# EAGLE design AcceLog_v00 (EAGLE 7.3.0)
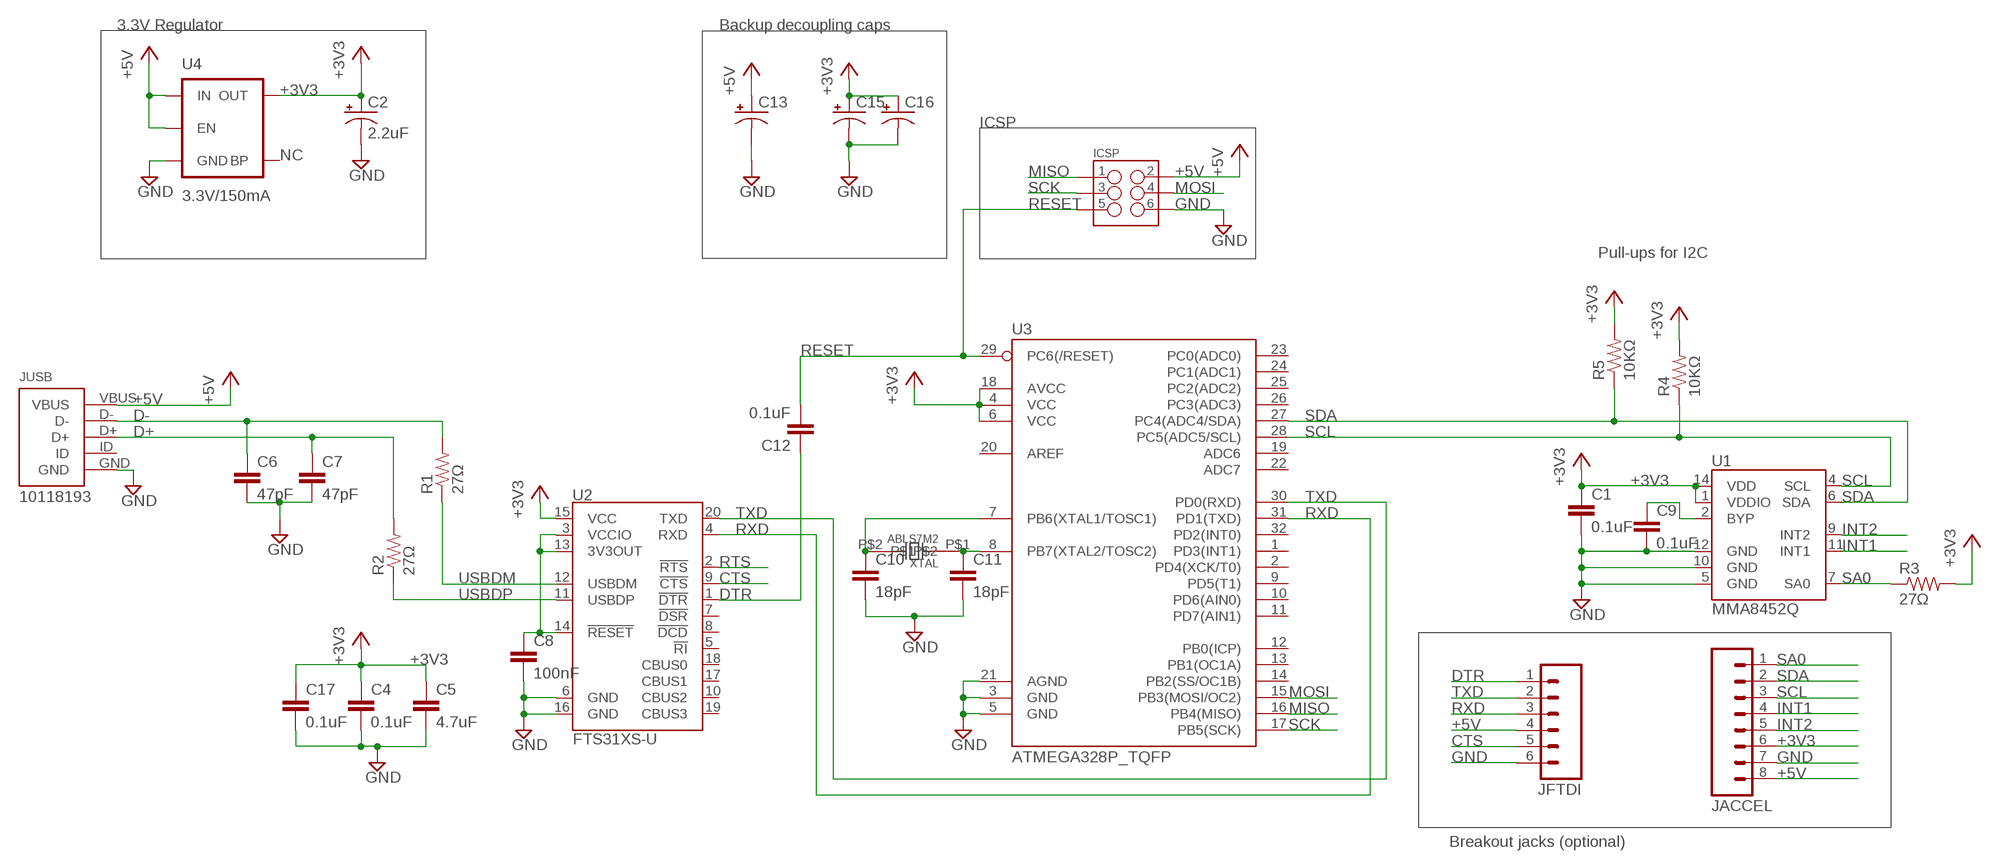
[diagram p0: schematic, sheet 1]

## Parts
C1  0.1uF  CAP0603-CAP  [0603-CAP]
C2  2.2uF  CAP_POL1206  [EIA3216]
C4  0.1uF  CAP0603-CAP  [0603-CAP]
C5  4.7uF  CAP0603-CAP  [0603-CAP]
C6  47pF  CAP0603-CAP  [0603-CAP]
C7  47pF  CAP0603-CAP  [0603-CAP]
C8  100nF  CAP0603-CAP  [0603-CAP]
C9  0.1uF  CAP0603-CAP  [0603-CAP]
C10  18pF  CAP0603-CAP  [0603-CAP]
C11  18pF  CAP0603-CAP  [0603-CAP]
C12  0.1uF  CAP0603-CAP  [0603-CAP]
C13  CPOL-USE2-5  [E2-5]
C15  CPOL-USE2-5  [E2-5]
C16  CPOL-USE2-5  [E2-5]
C17  0.1uF  CAP0603-CAP  [0603-CAP]
ICSP  M03X22X3_SILK_MALE_PTH  [2X3]
JACCEL  M08LOCK  [1X08_LOCK]
JFTDI  M06LOCK  [1X06_LOCK]
JUSB  10118193  [10118193]
R1  27Ω  RESISTOR0603-RES  [0603-RES]
R2  27Ω  RESISTOR0603-RES  [0603-RES]
R3  27Ω  RESISTOR0603-RES  [0603-RES]
R4  10KΩ  RESISTOR0603-RES  [0603-RES]
R5  10KΩ  RESISTOR0603-RES  [0603-RES]
U1  MMA8452Q  [QFN-16_0.5MM]
U2  FTS31XS-U  FT231XS  [SSOP20_L]
U3  ATMEGA328P_TQFP  [TQFP32-08]
U4  3.3V/150mA  V_REG_MIC52053.3V  [SOT23-5]
XTAL  ABLS7M2  [ABLS7M2]

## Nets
+3V3: C1.1 C2.A(+) C4.1 C5.1 C15.+ C16.+ C17.1 JACCEL.6 R3.2 R4.2 R5.2 U1.1(VDDIO) U1.14(VDD) U2.15(VCC) U3.4(VCC) U3.6(VCC) U3.18(AVCC) U4.5(OUT)
+5V: C13.+ ICSP.2 JACCEL.8 JFTDI.4 JUSB.VBUS U4.1(IN) U4.3(EN)
CTS: JFTDI.5 U2.9(!CTS)
D+: C7.1 JUSB.D+ R2.2
D-: C6.1 JUSB.D- R1.2
DTR: C12.1 JFTDI.1 U2.1(!DTR)
FTDI3V3: C8.1 U2.3(VCCIO) U2.13(3V3OUT) U2.14(!RESET)
GND: C1.2 C2.C(-) C4.2 C5.2 C6.2 C7.2 C8.2 C9.2 C10.2 C11.2 C13.- C15.- C16.- C17.2 ICSP.6 JACCEL.7 JFTDI.6 JUSB.GND U1.5(GND) U1.10(GND) U1.12(GND) U2.6(GND) U2.16(GND) U3.3(GND) U3.5(GND) U3.21(AGND) U4.2(GND)
INT1: JACCEL.4 U1.11(INT1)
INT2: JACCEL.5 U1.9(INT2)
MISO: ICSP.1 U3.16(PB4(MISO))
MOSI: ICSP.4 U3.15(PB3(MOSI/OC2))
N$10: C10.1 U3.7(PB6(XTAL1/TOSC1)) XTAL.P$2
N$11: C9.1 U1.2(BYP)
N$12: C11.1 U3.8(PB7(XTAL2/TOSC2)) XTAL.P$1
RESET: C12.2 ICSP.5 U3.29(PC6(/RESET))
RTS: U2.2(!RTS)
RXD: JFTDI.3 U2.4(RXD) U3.31(PD1(TXD))
SA0: JACCEL.1 R3.1 U1.7(SA0)
SCK: ICSP.3 U3.17(PB5(SCK))
SCL: JACCEL.3 R4.1 U1.4(SCL) U3.28(PC5(ADC5/SCL))
SDA: JACCEL.2 R5.1 U1.6(SDA) U3.27(PC4(ADC4/SDA))
TXD: JFTDI.2 U2.20(TXD) U3.30(PD0(RXD))
USBDM: R1.1 U2.12(USBDM)
USBDP: R2.1 U2.11(USBDP)
Unconnected: JUSB.ID U2.5(!RI) U2.7(!DSR) U2.8(!DCD) U2.10(CBUS2) U2.17(CBUS1) U2.18(CBUS0) U2.19(CBUS3) U3.1(PD3(INT1)) U3.2(PD4(XCK/T0)) U3.9(PD5(T1)) U3.10(PD6(AIN0)) U3.11(PD7(AIN1)) U3.12(PB0(ICP)) U3.13(PB1(OC1A)) U3.14(PB2(SS/OC1B)) U3.19(ADC6) U3.20(AREF) U3.22(ADC7) U3.23(PC0(ADC0)) U3.24(PC1(ADC1)) U3.25(PC2(ADC2)) U3.26(PC3(ADC3)) U3.32(PD2(INT0)) U4.4(BP)

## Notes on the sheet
- 3.3V Regulator | Backup decoupling caps
- ICSP
- NC
- Pull-ups for I2C
- Breakout jacks (optional)

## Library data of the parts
C1 C4-C12 C17 = SparkFun-Passives:CAP: Capacitor
C2 = SparkFun-Capacitors:CAP_POL: Capacitor Polarized
C13 C15 C16 = rcl:CPOL-US: POLARIZED CAPACITOR, American symbol
ICSP = SparkFun-Connectors:M03X2: 2x3 .1" header. Shrouded, with keying- CONN-10681 SMT- CONN-11415 Pogo pins- HW-11044; PROD_ID: CONN-09701
JACCEL = SparkFun-Connectors:M08: Header 8 Standard 8-pin 0.1" header. Use with straight break away headers (SKU : PRT-00116), right angle break away headers (PRT-00553), swiss pins (PRT-00743), machine pins (PRT-00117), and female headers (PRT-00115).
JFTDI = SparkFun-Connectors:M06: Header 6 Standard 6-pin 0.1" header. Use with straight break away headers (SKU : PRT-00116), right angle break away headers (PRT-00553), swiss pins (PRT-00743), machine pins (PRT-00117), and female headers (PRT-00115). Molex polarized connector foot print use with SKU : PRT-08094 with associated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
JUSB = MicroUSB:10118193: Micro USB B Jack for Surface Mount; MPN: 10118193; OC_DIGIKEY: 609-4616-1-ND; WEBSITE: http://www.digikey.com/product-detail/en/10118193-0001LF/609-4616-1-ND/2785380
R1-R5 = SparkFun-Passives:RESISTOR: Resistor
U1 = SparkFun-Sensors:MMA8452Q: MMA8452Q 3-Axis, 12/8-bit Digital Accelerometer Supply Voltage: 1.6-3.6V Range: +/- 2g, 4g, 8g Interface: I2C, 12-bit and 8-bit ODR: 1.56 Hz - 800 Hz Package: QFN-16 http://cache.freescale.com/files/sensors/doc/data_sheet/MMA8452Q.pdf; PROD_ID: IC-10769
U2 = SparkFun-DigitalIC:FT231X: FTDI FT231X Full Speed USB to Full-handshake UART This USB2.0 Full Speed IC offers a compact bridge to full handshake UART interfaces. The device is a UART, capable of operating up to 3MBaud, with low power consumption (8mA). The FT231X includes the complete FT-X series feature set and enables USB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; PROD_ID: IC-11524
U3 = SparkFun-DigitalIC:ATMEGA328P_TQFP; PROD_ID: IC-09069
U4 = SparkFun-PowerIC:V_REG_MIC5205: V_REG MIC5205 Standard 3.3V, 5V, and Adjustable 150mA LDO voltage regulator in SOT-23 layout. Micrel part MIC5205. BP (by-pass) pin is used to lower output noise with 470pF cap, may be left open. On the adjustable version BP is used to set output.; PROD_ID: VREG-00822
XTAL = AcceLogLib:ABLS7M2; DIGIKEY: 535-12830-1-ND; WEBSITE: http://www.digikey.com/product-detail/en/ABLS7M2-16.000MHZ-D-2Y-T/535-12830-1-ND/5135076

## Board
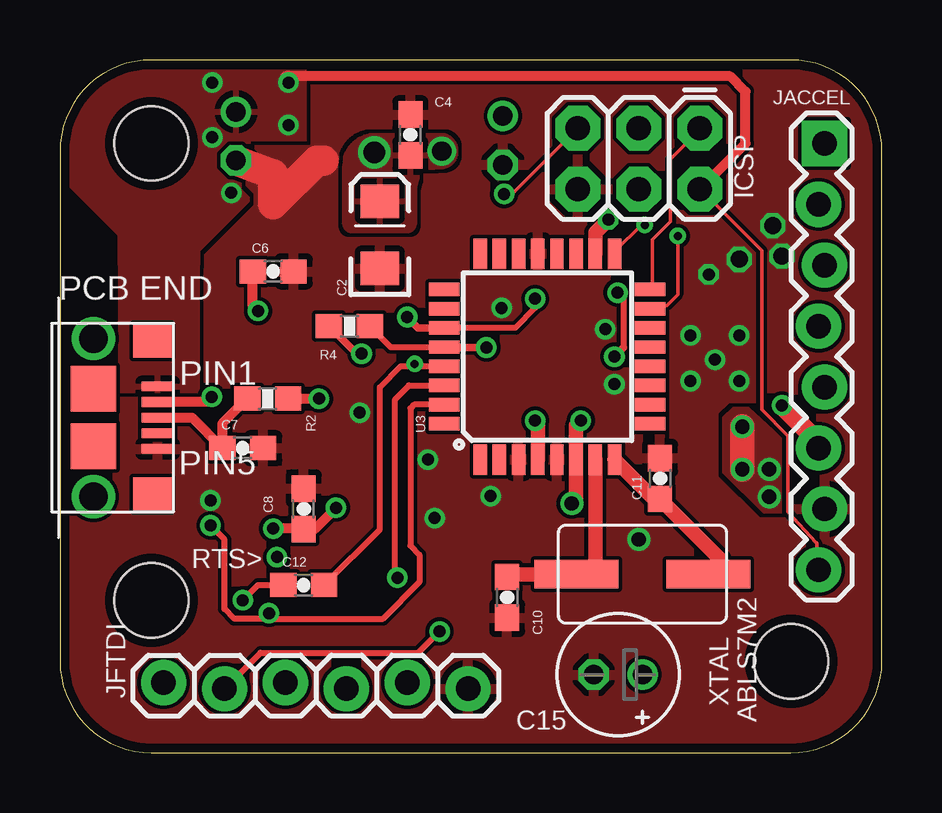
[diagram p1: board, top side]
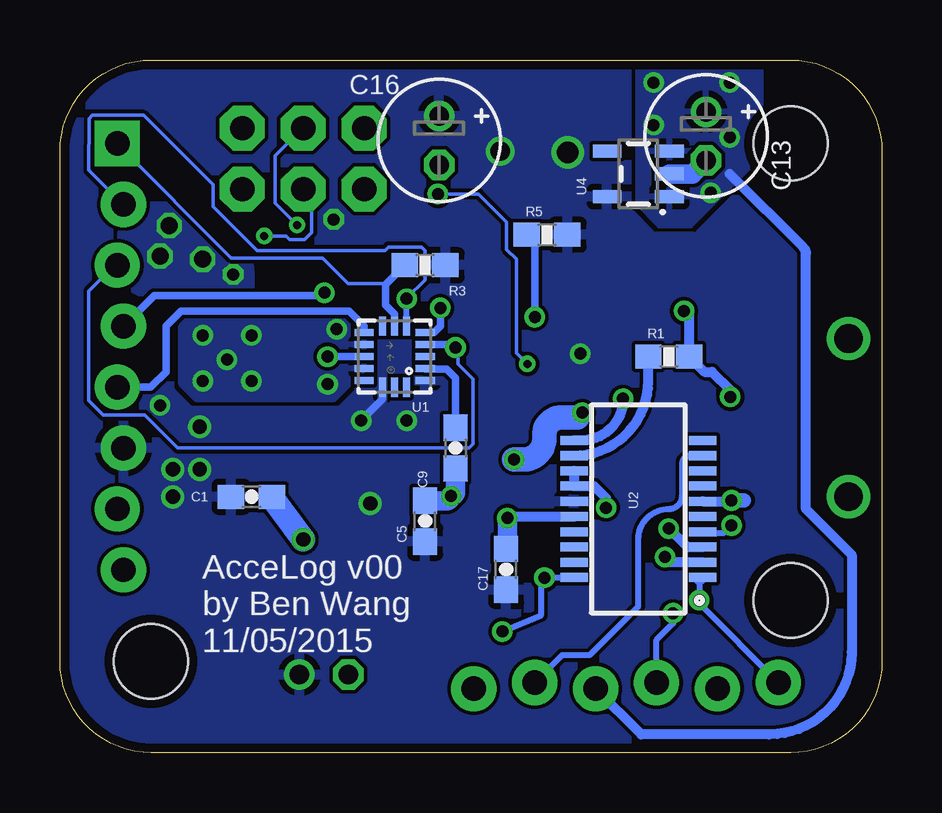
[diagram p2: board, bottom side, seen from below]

Size 34.27 x 28.88 mm. Coordinates in mm from the lower left corner, seen from the top.
Outline: 0,25.07 0,3.81 arc90 3.81,0 30.46,0 arc90 34.27,3.81 34.27,25.07 arc90 30.46,28.88 3.81,28.88 arc90 0,25.07
Copper layers (1*16): Top 0.0356mm / dielectric 1.5011mm / Bottom 0.0356mm
Design rules "LaenPCBOrder": minimum track width 6mil, minimum drill 13mil, track to track 6mil, track to pad 6mil, pad to pad 6mil, via to via 6mil, smd to smd 6mil, copper to edge 15mil, drill to drill 6mil, minimum pad ring 7mil, minimum via ring 7mil, stop-mask expansion 3mil, vias tented up to drill 0mil, thermal gap 10mil
Holes 3.1 mm at 30.48,3.81 3.81,25.4 3.81,6.35

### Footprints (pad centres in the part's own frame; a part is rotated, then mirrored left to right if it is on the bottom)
0603-CAP = smd 1.1 x 1: 1 -0.85,0; 2 0.85,0
EIA3216 = smd 1.4 x 1.6: A 1.4,0; C -1.4,0
E2-5 = drill 0.813 pad 1.27: + -1.016,0 | drill 0.813 pad 1.27 octagon: - 1.016,0
2X3 = drill 1.016 pad 1.88 octagon: 1 0,0; 2 0,2.54; 3 2.54,0; 4 2.54,2.54; 5 5.08,0; 6 5.08,2.54
1X08_LOCK = drill 1.016 pad 1.88 square: 1 0,0.127 | drill 1.016 pad 1.88: 2 2.54,-0.127; 3 5.08,0.127; 4 7.62,-0.127; 5 10.16,0.127; 6 12.7,-0.127; 7 15.24,0.127; 8 17.78,-0.127
1X06_LOCK = drill 1.016 pad 1.88: 1 0,0; 2 2.54,-0.254; 3 5.08,0; 4 7.62,-0.254; 5 10.16,0; 6 12.7,-0.254
10118193 = smd 0.4 x 1.35: D+ 0,2.675; D- -0.65,2.675; GND 1.3,2.675; ID 0.65,2.675; VBUS -1.3,2.675 | smd 1.4 x 1.6: P$6 -3.2,2.45; P$7 3.2,2.45 | smd 1.9 x 1.9: P$8 1.2,0; P$9 -1.2,0 | drill 1.2 pad 1.6: P$11 3.3,0; P$12 -3.3,0
0603-RES = smd 1.1 x 1: 1 -0.85,0; 2 0.85,0
QFN-16_0.5MM = smd 0.8 x 0.3: 1 -1.275,1; 2 -1.275,0.5; 3 -1.275,0; 4 -1.275,-0.5; 5 -1.275,-1; 9 1.275,-1; 10 1.275,-0.5; 11 1.275,0; 12 1.275,0.5; 13 1.275,1 | smd 0.3 x 0.8: 6 -0.5,-1.275; 7 0,-1.275; 8 0.5,-1.275; 14 0.5,1.275; 15 0,1.275; 16 -0.5,1.275
SSOP20_L = smd 0.381 x 1.143: 1 -2.857,-2.68; 2 -2.223,-2.68; 3 -1.587,-2.68; 4 -0.953,-2.68; 5 -0.318,-2.68; 6 0.318,-2.68; 7 0.953,-2.68; 8 1.587,-2.68; 9 2.223,-2.68; 10 2.857,-2.68; 11 2.857,2.68; 12 2.223,2.68; 13 1.587,2.68; 14 0.953,2.68; 15 0.318,2.68; 16 -0.318,2.68; 17 -0.953,2.68; 18 -1.587,2.68; 19 -2.223,2.68; 20 -2.857,2.68
TQFP32-08 = smd 1.27 x 0.559: 1 -4.293,2.8; 2 -4.293,2; 3 -4.293,1.2; 4 -4.293,0.4; 5 -4.293,-0.4; 6 -4.293,-1.2; 7 -4.293,-2; 8 -4.293,-2.8; 17 4.293,-2.8; 18 4.293,-2; 19 4.293,-1.2; 20 4.293,-0.4; 21 4.293,0.4; 22 4.293,1.2; 23 4.293,2; 24 4.293,2.8 | smd 0.559 x 1.27: 9 -2.8,-4.293; 10 -2,-4.293; 11 -1.2,-4.293; 12 -0.4,-4.293; 13 0.4,-4.293; 14 1.2,-4.293; 15 2,-4.293; 16 2.8,-4.293; 25 2.8,4.293; 26 2,4.293; 27 1.2,4.293; 28 0.4,4.293; 29 -0.4,4.293; 30 -1.2,4.293; 31 -2,4.293; 32 -2.8,4.293
SOT23-5 = smd 0.55 x 1.2: 1 -0.95,-1.3; 2 0,-1.3; 3 0.95,-1.3; 4 0.95,1.3; 5 -0.95,1.3
ABLS7M2 = smd 3.5 x 1.2: P$1 -2.75,0; P$2 2.75,0

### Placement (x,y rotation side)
C1  26.29,10.67 0 bottom
C2  13.34,21.59 90 top
C4  14.61,25.76 90 top
C5  19.05,9.65 90 bottom
C6  8.89,20.07 0 top
C7  7.62,12.7 0 top
C8  10.16,10.16 90 top
C9  17.78,12.7 270 bottom
C10  18.64,6.48 270 top
C11  25.02,11.43 90 top
C12  10.16,6.99 0 top
C13  7.34,25.7 270 bottom
C15  23.27,3.25 180 top
C16  18.47,25.53 270 bottom
C17  15.67,7.65 90 bottom
ICSP  26.67,26.04 180 top
JACCEL  31.75,25.4 270 top
JFTDI  4.32,2.92 0 top
JUSB  1.4,13.97 270 top
R1  8.89,16.51 0 bottom
R2  8.66,14.76 180 top
R3  19.05,20.32 0 bottom
R4  12.06,17.78 180 top
R5  13.97,21.59 0 bottom
U1  20.32,16.51 180 bottom
U2  10.16,10.16 90 bottom
U3  20.32,16.51 90 top
U4  10.16,24.13 90 bottom
XTAL  24.28,7.44 180 top

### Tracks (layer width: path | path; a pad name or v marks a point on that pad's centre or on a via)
+3V3  (via drill 0.5, 0.6, 0.8, 0.9)
  Top 0.305: R4.2 12.36,16.64 v12.57,16.64
  Top 0.61: U3.4 19.92,13.61 v19.81,13.84 | U3.6 21.52,13.65 v21.72,13.84 | v22.86,22.23 22.32,21.68 U3.18 | v21.34,10.39 21.51,10.57 21.51,12.6
  Top 0.813: 31.5,12.7 31.5,13.08 v30.1,14.48
  Top 1.016: 31.5,12.7 31.75,12.7 | v28.45,13.59 v28.45,11.81
  Bottom 0.305: U1.14 20.82,14.74 v21.72,13.84
  other vias: 13.11,25.02 15.91,25.08 29.57,10.67 29.57,11.81
  pour Bottom (rank 5): 0,30.48 36.83,30.48 36.83,-5.08 0,-5.08
  pour Top: 27.69,13.97 28.07,14.35 28.7,14.35 30.23,12.95 30.23,10.16 30.1,10.03 29.34,10.03 27.69,11.68
  pour Top: 11.89,23.11 11.89,24.46 arc-90 13.16,25.73 15.85,25.73 arc-90 16.48,25.1 16.48,25.07 arc-90 15.85,24.43 15.7,24.43 arc90 14.76,23.5 14.76,22.15 14.76,22.09 arc-90 14.44,21.77 13.06,21.77 12.2,21.77 arc-90 11.89,22.09
+5V  (via drill 0.5)
  Top 0.152: JACCEL.8 31.55,7.67 31.55,8.74 31.52,8.74 30.35,10.03 30.35,13.21 29.26,14.3 29.26,20.93 26.82,23.37 ICSP.2
  Top 0.406: ICSP.2 28.57,25.4 28.57,27.56 27.94,28.19 9.4,28.19
  Bottom 0.406: JFTDI.4 10.03,0.76 4.7,0.76 arc-90 1.27,4.19 1.27,8.26 3.17,10.16 3.17,20.82 arc-45 3.27,21.05 6.35,24.13
  other vias: 6.35,25.65 9.53,26.16 9.53,27.94 6.35,27.94 7.14,23.34
  pour Bottom (rank 3): 5.08,25.4 4.57,25.4 8,21.97 9.27,21.97 10.16,22.86 10.16,31.75 5.08,31.75
  pour Top (rank 3): 2.54,15.11 5.71,15.11 5.71,21.16 2.54,21.16
  pour Top (rank 2): 2.54,20.32 2.54,21.92 5.08,24.46 5.08,29.21 6.35,29.21 10.16,29.21 10.16,25.4 5.71,20.95 5.71,20.68 5.71,20.32
  pour Top (rank 3): 2.54,21.59 -1.27,25.4 -1.27,26.67 1.27,29.21 5.08,29.21 6.35,27.94 6.35,24.13 3.81,21.59
CTS
  Bottom 0.254: JFTDI.5 13.34,4.06 12.19,4.06 10.16,6.1 10.16,8.89 arc90 8.89,10.16 arc-90 8.33,10.72 8.33,12.04 arc90 7.99,12.38 U2.9 | 7.66,12.38 U2.9 | 7.81,12.38 U2.9
D+
  Top 0.406: JUSB.D+ 5.5,13.97 C7.1 6.77,13.72 R2.2
D-  (via drill 0.5)
  Top 0.406: v8.26,18.41 8.04,18.63 C6.1 | v6.33,14.83 6.11,14.62 JUSB.D-
  Bottom 0.406: v8.26,18.41 8.04,18.2 R1.2 7.41,15.88 7.09,15.88 6.33,15.11 v6.33,14.83
DTR  (via drill 0.5)
  Top 0.254: v7.62,6.35 8.26,6.99 C12.1
  Bottom 0.254: 7.62,7.16 v7.62,6.35 | 7.62,6.22 JFTDI.1
  Bottom 0.406: U2.1 7.62,7.16 | v7.62,6.35 7.62,6.22
FTDI3V3  (via drill 0.5)
  Top 0.406: v11.51,10.21 10.61,9.31 C8.1 | 10.15,9.3 10.1,9.35 v8.89,9.35
  Top 0.813: 10.2,9.27 arc-90 C8.1 arc-90 10.15,9.3
  Bottom 0.406: U2.13 U2.14 12,11.11 11.51,10.62 v11.51,10.21 | v8.89,9.35 8.12,8.57 U2.3
GND  (via drill 0.5, 0.6, 0.7)
  Top 0.813: 11,24.69 11,24.77
  Top 1.27: 11,24.69 10.72,24.69 8.89,22.86 8.89,24.1 U4.2 C13.-
  Bottom 0.305: v18.41,18.54 18.41,17.78 18.68,17.51 U1.5
  Bottom 0.406: v15.62,9.78 15.56,9.84 U2.16 | U2.6 6.31,10.48 v6.27,10.52
  Bottom 0.61: 5.75,10.52 v6.27,10.52
  Bottom 0.813: C13.- 7.9,24.13 U4.2 | C17.2 15.62,8.55 v15.62,9.78 | C9.2 17.78,10.92 arc90 v17.96,10.69 arc90 18.2,10.5 C5.2
  Bottom 1.016: v24.13,8.89 C1.2 | 12.7,13.97 13.39,13.97 arc-90 14.07,13.28 14.07,13.11 arc90 14.96,12.22 v15.34,12.22
  other vias: 27.3,16.38 28.32,17.4 26.29,15.49 26.29,17.4 27.05,19.94 28.32,20.57 29.72,21.97 30.1,20.7 28.32,15.49 23.11,15.37 22.73,17.65 12.5,14.17
  pour Top (rank 5): -1.27,31.75 35.56,31.75 35.56,-2.54 -1.27,-2.54
  pour Bottom: 22.86,18.41 21.59,17.14 21.59,16 22.86,14.73 28.57,14.73 29.21,15.37 29.21,17.78 28.57,18.41
  pour Bottom: 26.67,19.05 30.48,19.05 arc90 31.75,20.32 31.75,21.59 arc90 30.48,22.86 29.21,22.86 arc90 26.29,19.94 26.29,19.43 arc90
  pour Top: 7.67,25.22 11.43,25.22 8.46,22.25 8.46,23.09 7.8,23.75 8.2,24.16 8.2,24.99
INT1  (via drill 0.5)
  Top 0.254: v23.24,19.18 23.5,18.92 23.5,16.89
  Top 0.305: 23.5,16.89 v23.11,16.51
  Bottom 0.305: U1.11 v23.11,16.51 | JACCEL.4 30.35,19.05 23.24,19.05 v23.24,19.18
INT2
  Bottom 0.305: U1.9 21.59,17.79 22.23,18.41 29.21,18.41 29.84,17.78 29.84,15.88 30.48,15.24 JACCEL.5
MISO
  Top 0.152: U3.16 24.69,19.41 24.69,21.39 25.45,22.15 25.45,24.74 26.67,25.96 ICSP.1
MOSI  (via drill 0.33)
  Top 0.152: v25.76,21.54 25.76,19.1 25.3,18.64 24.69,18.64 U3.15
  Bottom 0.152: v25.76,21.54 24.84,21.54 24.69,21.39 24.08,21.39 23.77,21.69 23.77,23.06 24.08,23.37 ICSP.4
N$10
  Top 0.61: U3.7 22.32,7.72 XTAL.P$2 18.76,7.44 C10.1
N$11
  Bottom 0.305: U1.2 19.04,16 18.16,16 17.78,15.62 C9.1
N$12
  Top 0.152: 23.16,12.09 U3.8
  Top 0.61: U3.8 24.76,10.58 C11.1 27.54,8.06 XTAL.P$1
RESET  (via drill 0.33, 0.5)
  Top 0.152: v14.78,16.2 14.78,16.11 | v18.52,23.29 18.85,23.29 ICSP.5
  Top 0.254: C12.2 13.34,9.31 13.34,15.24 14.21,16.11 14.78,16.11 U3.29
  Bottom 0.152: v14.78,16.2 15.24,16.66 15.24,20.57 15.65,20.98 15.65,22.12 16.82,23.29 v18.52,23.29
RTS  (via drill 0.5)
  Bottom 0.406: U2.2 8.83,7.94 v9.04,8.15
RXD  (via drill 0.5)
  Top 0.254: U3.31 14.76,14.51 14.61,14.35 14.61,8.64 14.99,8.26 14.99,7.11 13.46,5.59 8.94,5.59 v8.71,5.82 8.48,5.59 7.26,5.59 6.86,5.99 6.86,8.89 v6.27,9.47
  Bottom 0.254: JFTDI.3 9.4,4.7 8.71,5.38 v8.71,5.82 | U2.4 7.44,9.17 6.58,9.17 v6.27,9.47
SA0
  Bottom 0.152: 20.69,19.53 20.73,19.56 22.25,19.56 23.32,20.62 27.13,20.62 31.85,25.35 JACCEL.1
  Bottom 0.305: U1.7 20.32,18.29 20.7,18.67 20.7,19.52 20.69,19.53 R3.1
SCK  (via drill 0.33)
  Top 0.152: v24.38,22 24.23,22 23.16,20.93 U3.17
  Bottom 0.152: v24.38,22 25.3,22.91 25.3,24.89 24.23,25.96 ICSP.3
SCL  (via drill 0.5)
  Top 0.254: R4.1 13.79,16.91 U3.28
  Top 0.305: v17.78,16.89 16.05,16.89 U3.28
  Bottom 0.152: v17.78,16.89 17.68,16.82 17.68,16.2 17.04,15.57 17.04,12.88 17.22,12.7 29.36,12.7 30.73,14.07 32.46,14.07 33.07,14.68 33.07,19.25 32,20.32 JACCEL.3
  Bottom 0.305: U1.4 17.9,17.01 v17.78,16.89
SDA  (via drill 0.5)
  Top 0.254: v19.81,18.92 19.81,18.54 18.98,17.71 U3.27
  Top 0.305: v14.48,18.16 14.93,17.71 U3.27
  Bottom 0.152: JACCEL.2 31.7,22.91 33.07,24.28 33.05,26.44 32.92,26.57 30.79,26.57 27.89,23.67 27.89,22.76 26.06,20.93 20.73,20.93 20.57,21.08 19.2,21.08 19.05,20.93 19.05,19.71 19.81,18.95 v19.81,18.92
  Bottom 0.254: U1.6 19.82,18.79 v19.81,18.92
  Bottom 0.305: R5.1 arc90 14.48,21.25 v14.48,18.16
TXD  (via drill 0.5)
  Top 0.254: U3.30 14.55,15.31 13.97,14.73 13.97,7.39 v14.07,7.29 | JFTDI.2 8.36,4.17 14.94,4.17 v15.82,5.05 15.67,4.9
  Bottom 0.254: v15.82,5.05 14.22,5.71 14.22,7.14 v14.07,7.29 12.85,7.29 U2.20
USBDM
  Bottom 0.406: U2.12 arc-90 9.74,15.48 R1.1
USBDP  (via drill 0.5)
  Top 0.406: R2.1 v10.79,14.76
  Bottom 0.406: v10.79,14.76 arc90 12.54,13.02 U2.11

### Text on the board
tNames: RTS>
bNames: AcceLog v00 / by Ben Wang / 11/05/2015

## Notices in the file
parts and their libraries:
SparkFun-Sensors: Licensing: Creative Commons ShareAlike 4.0 International - https://creativecommons.org/licenses/by-sa/4.0
